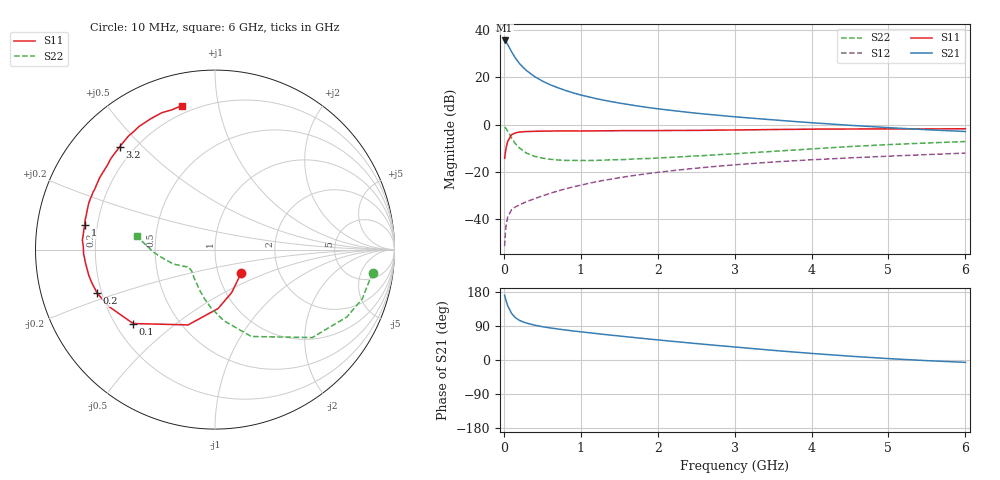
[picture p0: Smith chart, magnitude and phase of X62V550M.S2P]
! SIEMENS Small Signal Semiconductors
! BFP193W
! Si NPN RF Bipolar Junction Transistor in SOT343
! VCE = 2.5 V  IC = 50 mA
! Common Emitter S-Parameters:  April 1994
# GHz  S  MA  R  50
!  f  S11  S21  S12  S22
! GHz  MAG  ANG  MAG  ANG  MAG  ANG  MAG  ANG
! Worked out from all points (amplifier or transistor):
!   40 points, 10 MHz to 6 GHz, reference 50 ohm
!   highest |S21| = 35.7 dB at 10 MHz (marker M1)
!   |S21| within 3 dB of that: start of sweep to 71.19 MHz
!   unconditionally stable (mu >= 1): 544.6 MHz to 3.946 GHz
!   at 200 MHz: K = 0.61, MSG = 30.0 dB, |S12| = -34.0 dB
!   at 1.5 GHz: K = 1.14, MAG = 13.5 dB, |S12| = -22.4 dB
!   at 6 GHz: K = 0.95, MSG = 4.6 dB, |S12| = -12.0 dB
!   S11 on the Smith chart (normalised r, x): 10 MHz: 1.29, -0.34; 100 MHz: 0.27, -0.36; 200 MHz: 0.18, -0.17; 1 GHz: 0.15, +0.09; 3.2 GHz: 0.15, +0.43; 6 GHz: 0.16, +0.78
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0.01  0.1949 -41.0  60.66 170.9  0.0027 82.9  0.8871 -8.3
0.02  0.2567 -68.7  59.27 163.5  0.0052 73.6  0.8654 -18.4
0.03  0.3289 -87.0  56.66 156.0  0.0076 72.0  0.8253 -27.0
0.05  0.4456 -109.7  49.88 143.1  0.0111 61.3  0.7309 -42.1
0.1  0.6145 -137.9  35.04 122.9  0.0159 48.7  0.5248 -67.3
0.15  0.6721 -152.0  25.73 111.6  0.0183 45.0  0.3989 -83.0
0.2  0.6996 -159.7  20.02 105.0  0.02 45.7  0.3255 -93.9
0.25  0.7115 -165.1  16.39 100.5  0.0219 46.7  0.2809 -101.9
0.3  0.7178 -168.6  13.76 97.1  0.0238 48.5  0.2486 -108.9
0.4  0.7255 -174.2  10.45 91.9  0.0273 52.3  0.2147 -118.6
0.5  0.7327 -178.3  8.424 87.9  0.0312 55.3  0.197 -125.9
0.6  0.7338 178.7  7.035 84.7  0.0353 57.7  0.1863 -131.5
0.7  0.741 175.9  6.083 81.9  0.0397 59.4  0.1794 -135.4
0.8  0.7384 173.3  5.316 79.2  0.0439 61.0  0.1761 -138.1
1  0.7374 169.3  4.256 74.4  0.0526 62.2  0.1756 -142.8
1.1  0.7421 167.3  3.899 72.1  0.0575 62.7  0.1753 -144.3
1.6  0.7501 158.1  2.707 61.2  0.0803 62.4  0.1844 -148.7
2.2  0.757 148.2  1.992 49.1  0.1072 59.5  0.2053 -154.0
3.2  0.7812 132.7  1.387 30.8  0.1502 52.3  0.2554 -163.3
4.5  0.8125 116.0  0.973 10.1  0.1991 42.4  0.3462 -178.1
5.5  0.8148 107.2  0.784 -1.7  0.2335 35.5  0.411 173.3
6  0.8231 103.1  0.72 -6.2  0.2516 32.5  0.4413 170.1
